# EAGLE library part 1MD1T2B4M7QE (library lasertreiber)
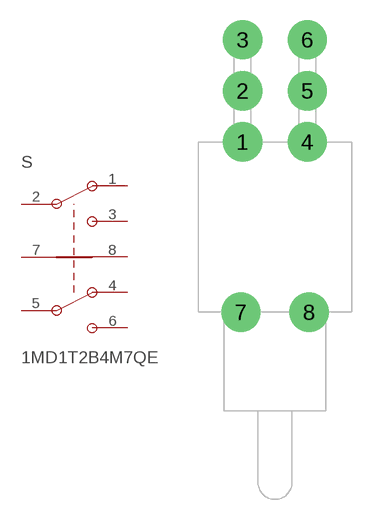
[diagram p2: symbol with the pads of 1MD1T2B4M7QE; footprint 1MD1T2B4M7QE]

Designator prefix S

## 1MD1T2B4M7QE  [1MD1T2B4M7QE]
1  A1
2  A
3  A2
4  B1
5  B
6  B2
7  GND
8  GND

## Footprint 1MD1T2B4M7QE (pad centres in mm)
drill 1.95: 1 -2.413,0; 2 -2.413,3.81; 3 -2.413,7.62; 4 2.413,0; 5 2.413,3.81; 6 2.413,7.62; 7 -2.54,-12.7; 8 2.54,-12.7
